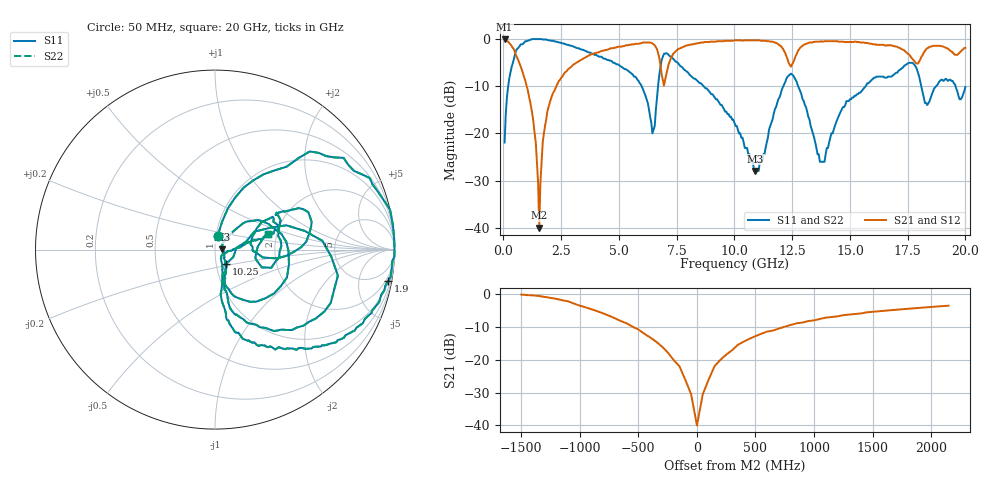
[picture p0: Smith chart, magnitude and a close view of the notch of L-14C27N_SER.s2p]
# MHZ S MA R 50
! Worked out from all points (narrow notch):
!   400 points, 50 MHz to 20 GHz, reference 50 ohm
!   highest |S21| = -0.09 dB at 50 MHz (marker M1); lowest = -40.0 dB at 1.55 GHz (marker M2)
!   notch at M2: 38.6 dB deep, 364 MHz wide at half that depth
!   lowest |S11| = -28.0 dB at 10.9 GHz (marker M3), VSWR 1.08, Z = 54.2 + j0.22 ohm
!   |S11| at or under -10 dB: 5.984 GHz to 6.693 GHz (709.2 MHz wide, 11.2 % of centre); 8.669 GHz to 12.12 GHz (3.447 GHz wide, 33.2 % of centre); 12.76 GHz to 15.68 GHz (2.922 GHz wide, 20.5 % of centre)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
!   |S22| runs from -28.0 to 0.0 dB; largest |S21 - S12| = 0
!   S11 on the Smith chart (normalised r, x): 50 MHz: 1.02, +0.16; 1.9 GHz: 1, -11; 10.25 GHz: 1.11, -0.18; 20 GHz: 1.80, +0.35
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50  0.08 78.7  0.99 -3.5  0.99 -3.5  0.08 78.7
350  0.5 57.1  0.85 -29.2  0.85 -29.2  0.5 57.1
1200  0.99 14.5  0.19 -77.8  0.19 -77.8  0.99 14.5
1400  1 6.9  0.08 -80.8  0.08 -80.8  1 6.9
1550  1 1.3  0.01 19.5  0.01 19.5  1 1.3
1700  0.99 -3.7  0.08 77.2  0.08 77.2  0.99 -3.7
1900  0.98 -10.4  0.17 75.1  0.17 75.1  0.98 -10.4
3400  0.77 -44.8  0.61 46.0  0.61 46.0  0.77 -44.8
5750  0.39 -80.6  0.89 14.2  0.89 14.2  0.39 -80.6
6450  0.1 -49.1  0.9 -5.7  0.9 -5.7  0.1 -49.1
6700  0.33 21.6  0.7 -22.7  0.7 -22.7  0.33 21.6
6950  0.7 -12.0  0.32 5.3  0.32 5.3  0.7 -12.0
7350  0.62 -46.3  0.7 26.7  0.7 26.7  0.62 -46.3
10050  0.12 -61.6  0.97 -5.8  0.97 -5.8  0.12 -61.6
10250  0.1 -52.9  0.97 -7.4  0.97 -7.4  0.1 -52.9
10900  0.04 2.9  0.97 -13.0  0.97 -13.0  0.04 2.9
12450  0.43 -21.1  0.51 -16.6  0.51 -16.6  0.43 -21.1
13350  0.11 -67.6  0.92 -11.7  0.92 -11.7  0.11 -67.6
13900  0.05 -22.7  0.95 -18.4  0.95 -18.4  0.05 -22.7
14850  0.22 13.0  0.93 -27.0  0.93 -27.0  0.22 13.0
16700  0.4 30.5  0.86 -39.9  0.86 -39.9  0.4 30.5
20000  0.31 16.7  0.81 -44.7  0.81 -44.7  0.31 16.7
